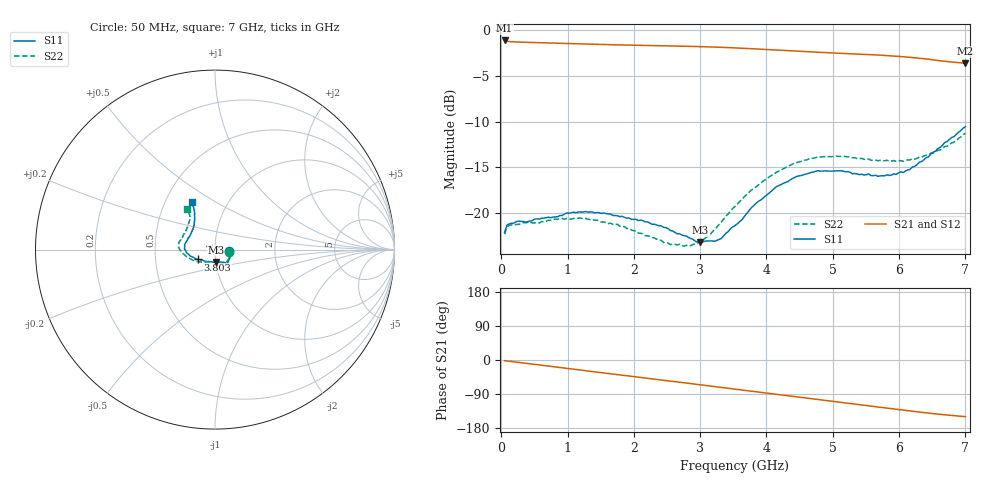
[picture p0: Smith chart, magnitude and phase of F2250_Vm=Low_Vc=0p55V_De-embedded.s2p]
! Integrated Device Technology
! Corporate Headquarters
! 6024 Silver Creek Valley Road
! San Jose, CA 95138  USA
! Phone:  1-408-284-8200
! Toll Free:  1-800-223-1366
! Webpage:  http://www.idt.com/
! Timing and RF Division
! 515 Groton Road, Suite 102
! Westford, MA 01886-6024
! Device:  F2250
! Description: Voltage Variable RF Attenuator
! Frequency:  50.0 -  6000.00 MHz
! Package:  3x3 mm Thin QFN Plastic Package: 16 pin
! Ports:  2 RF, 3 DC
!  Pin  1  = GND
!  Pin  2  = NC
!  Pin  3  = RF1  = Port 1
!  Pin  4  = NC
!  Pin  5  = GND
!  Pin  6  = GND
!  Pin  7  = GND
!  Pin  8  = GND
!  Pin  9  = NC
!  Pin 10  = RF2  = Port 2
!  Pin 11  = NC
!  Pin 12  = GND
!  Pin 13  = GND
!  Pin 14  = VCNTRL
!  Pin 15  = VDD
!  Pin 16  = VMODE
! Vcntrl:  0.550 Volts
! Vmode:  +0.000 Volts
! Vdd:  +3.30  Volts
! Current:  1.134 mA
! Data:  The device was measured on a the F2250 evaluation board which has
!  individual transmission lines to the RF pins.  Data was collected
!  using a calibrated network analyzer.  The evaluation board was
!  de-embedded using a TRL calibration technique.
!  The reference plane is the edge of the package pin.
! Misc:  SN 10
!  Action Tracker AT0258
! Date Measured:  2014-11-26
! Date:  2015-10-15  MJV
! Note:
!  Integrated Device Technology supplies this data as a sample of measured
!  data at the package pin for this product.  Your particular data for this
!  product may vary.
!  Data was taken at 25 degrees C.
!  Integrated Device Technology reserves the right to change this data at anytime.
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# GHz S dB R 50
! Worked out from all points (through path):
!   201 points, 50 MHz to 7 GHz, reference 50 ohm
!   highest |S21| = -1.15 dB at 50 MHz (marker M1); lowest = -3.6 dB at 7 GHz (marker M2)
!   group delay of S21, straight-line fit = 60.1 ps
!   lowest |S11| = -23.2 dB at 3.004 GHz (marker M3), VSWR 1.15, Z = 50.2 - j6.96 ohm
!   |S11| at or under -10 dB: start of sweep to end of sweep
!   |S22| runs from -23.6 to -11.3 dB; largest |S21 - S12| = 0.00042
!   S11 on the Smith chart (normalised r, x): 50 MHz: 1.17, -0.02; 3.803 GHz: 0.82, -0.09; 7 GHz: 0.68, +0.40
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0.05  -22.08 -7.0  -1.15 -1.8  -1.15 -1.8  -22.29 -8.0
0.08475  -21.31 -7.0  -1.24 -2.5  -1.24 -2.5  -21.47 -7.5
0.15425  -21.09 -9.1  -1.29 -4.0  -1.29 -4.0  -21.27 -9.4
0.6755  -20.49 -29.4  -1.42 -15.4  -1.42 -15.4  -20.90 -32.4
1.2315  -19.89 -47.1  -1.54 -27.4  -1.54 -27.4  -20.60 -54.3
1.75275  -20.28 -53.9  -1.64 -38.5  -1.63 -38.5  -21.21 -63.5
2.37825  -21.36 -56.2  -1.72 -51.8  -1.72 -51.8  -22.92 -70.8
2.7605  -22.46 -67.5  -1.78 -60.2  -1.78 -60.2  -23.60 -87.6
3.00375  -23.18 -84.3  -1.83 -65.6  -1.82 -65.6  -23.04 -106.0
3.14275  -23.02 -95.5  -1.86 -68.6  -1.85 -68.6  -22.39 -117.5
3.3165  -22.77 -113.9  -1.90 -72.5  -1.90 -72.5  -20.99 -129.2
3.525  -21.36 -131.7  -1.96 -77.2  -1.97 -77.2  -19.27 -141.4
3.803  -19.20 -150.0  -2.07 -83.3  -2.07 -83.3  -17.32 -154.1
4.1505  -17.10 -164.4  -2.21 -91.0  -2.21 -91.0  -15.53 -168.0
4.4285  -16.09 -173.1  -2.31 -97.0  -2.31 -97.0  -14.53 -175.7
4.7065  -15.50 179.6  -2.42 -103.0  -2.42 -103.0  -14.01 178.0
5.15825  -15.41 168.6  -2.58 -112.7  -2.58 -112.7  -13.77 168.3
5.85325  -15.88 144.9  -2.82 -127.6  -2.83 -127.7  -14.33 152.7
6.166  -15.22 133.0  -2.99 -134.4  -2.99 -134.5  -14.19 143.6
6.444  -13.85 123.5  -3.20 -140.2  -3.20 -140.3  -13.66 134.1
6.82625  -11.65 116.9  -3.52 -146.9  -3.52 -146.9  -12.27 125.9
7  -10.56 116.0  -3.64 -149.6  -3.64 -149.6  -11.28 124.4
